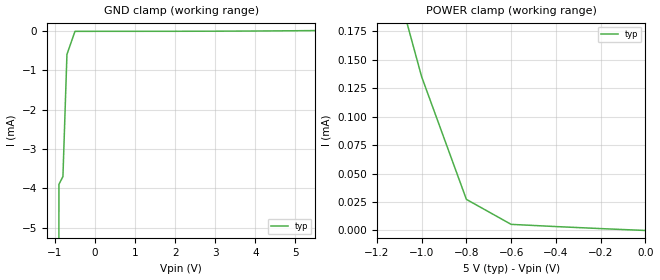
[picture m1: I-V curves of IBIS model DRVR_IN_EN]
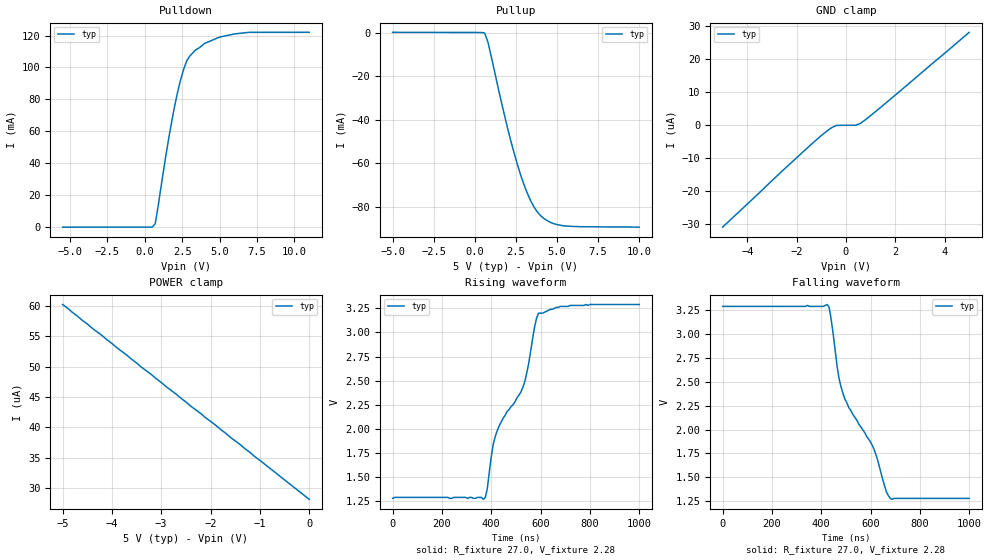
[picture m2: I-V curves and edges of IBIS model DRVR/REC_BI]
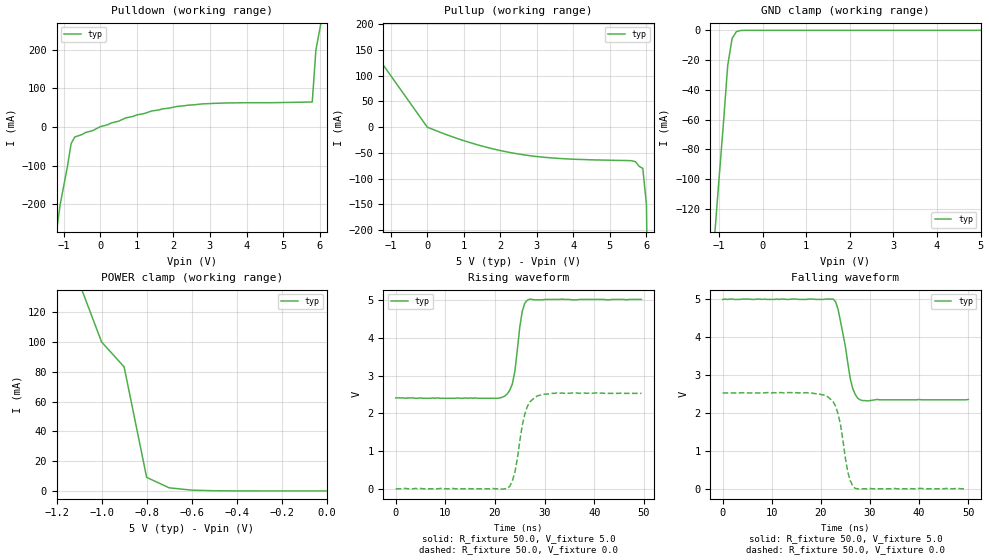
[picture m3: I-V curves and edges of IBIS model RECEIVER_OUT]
|   Texas Instruments Incorporated
|   Data Transmissions Products
|   IBIS Model for SN65HVD1786
|   SOIC 8-pin (D), PDIP 8-pin (P), VCC=5V
[IBIS Ver]   3.2
[Comment char]   |_char
[File name]   sllc356.ibs
[File Rev]   1.0
[Date]   6Aug08
[Source]   File originated at Texas Instruments Incorporated.
   Data Transmission Products Group.
[Notes]
[Disclaimer]
(C) Copyright Texas Instruments Incorporated 2002
   All rights reserved
  Texas Instruments Incorporated hereby grants the user of this IBIS
model a non-exclusive, nontransferable license to use this IBIS model
under the following terms.  Before using this IBIS model, the user
should read this license.  If the user does not accept these terms,
the IBIS model should be returned to Texas Instruments within 30 days.
  The user is granted this license only to use the IBIS model and
is not granted rights to sell, load, rent, lease or license the IBIS
model in whole or in part, or in modified form to anyone other than
user.  User may modify the IBIS model to suit its specific applications
but rights to derivative works and such modifications shall belong to
Texas Instruments.
  This IBIS model is provided on an "AS IS" basis and Texas Instruments
makes absolutely no warranty with respect to the information contained
herein.  TEXAS INSTRUMENTS DISCLAIMS AND CUSTOMER WAIVES ALL WARRANTIES,
EXPRESS OR IMPLIED, INCLUDING WARRANTIES OF MERCHANTABILITY OR FITNESS
FOR A PARTICULAR PURPOSE. The entire risk as to quality and performance
is with the Customer. ACCORDINGLY, IN NO EVENT SHALL THE COMPANY BE LIABLE
FOR ANY DAMAGES, WHETHER IN CONTRACT OR TORT,INCLUDING ANY LOST PROFITS
OR OTHER INCIDENTAL, CONSEQUENTIAL, EXEMPLARY, OR PUNITIVE DAMAGES ARISING
OUT OF THE USE OR APPLICATION OF THE IBIS model provided in this package.
Further, Texas Instruments reserves the right to discontinue or make changes
without notice to any product herein to improve reliability, function, or
design. Texas Instruments does not convey any license under patent rights
or any other intellectual property rights, including those of third parties.
Contact Texas Instruments at ATTN:DATA TRANSMISSIONS
[Copyright]   Copyright 2002, Texas Instruments, All Rights Reserved
[Component]   HVD1786_D
[Manufacturer]  Texas Instruments Incorporated
[Package]
|   typ   min   max
R_pkg   0.1017   0.0608   0.1359
L_pkg   1.9890nH   1.6927nH   2.3143nH
C_pkg   0.3794pF   0.3519pF   0.3977pF
[Pin]   signal_name   model_name   R_pin   L_pin   C_pin
1   R   RECEIVER_OUT   0.108   1.993n   0.363p
2   REB   DRVR_IN_EN   0.103   1.929n   0.373p
3   DE   DRVR_IN_EN   0.103   1.932n   0.373p
4   D   DRVR_IN_EN   0.107   2.016n   0.352p
5   GND   GND   0.064   1.778n   0.394p
6   A   DRVR/REC_BI   0.131   2.258n   0.391p
7   B   DRVR/REC_BI   0.136   2.314n   0.391p
8   VCC   POWER   0.061   1.693n   0.398p
[Diff_pin]   inv_pin   vdiff   tdelay_typ   tdelay_min   tdelay_max
| The 'A' pin is Diff_pin and the 'B' pin is the inv_pin
6   7   0.200   0   0   0
[Component]   HVD1786_P
[Manufacturer]  Texas Instruments Incorporated
[Package]
|   typ   min   max
R_pkg   0.0833   0.0374   0.1222
L_pkg   2.7019nH   1.3887nH   3.6744nH
C_pkg   0.6414pF   0.3892pF   0.8943pF
[Pin]   signal_name   model_name   R_pin   L_pin   C_pin
1   R   RECEIVER_OUT   0.078   3.269n   0.675p
2   REB   DRVR_IN_EN   0.100   2.510n   0.648p
3   DE   DRVR_IN_EN   0.111   2.858n   0.640p
4   D   DRVR_IN_EN   0.074   2.765n   0.640p
5   GND   GND   0.037   1.389n   0.389p
6   A   DRVR/REC_BI   0.105   3.674n   0.894p
7   B   DRVR/REC_BI   0.122   2.925n   0.663p
8   VCC   POWER   0.038   2.226n   0.583p
[Diff_pin]   inv_pin   vdiff   tdelay_typ   tdelay_min   tdelay_max
| The 'A' pin is Diff_pin and the 'B' pin is the inv_pin
6   7   0.200   0   0   0
| Models and submodels in the file (3): DRVR_IN_EN (Input), DRVR/REC_BI (I/O), RECEIVER_OUT (3-state)
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|   Driver Input / Receiver Enable Model
[Model]   DRVR_IN_EN
Model_type   Input
|Signals   D,DE,RE
Vinh = 2.0
Vinl = 0.8
|   typ   min   max
C_comp   1.0pF   NA   NA
|   typ   min   max
[Temperature Range]   25.0   -40   105
[Voltage range]   5.0V   4.5V   5.5V
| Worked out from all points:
|   GND clamp passes 1 mA (typ) near -0.71 V on its own axis
|   POWER clamp passes 1 mA (typ) near -2.08 V on its own axis
[GND_clamp]
|   Voltage   I(typ)   I(min)   I(max)
-5.5V     -8.7A      NA         NA
-2V       -1.9A      NA         NA
-900mV    -3.9mA     NA         NA
-800mV    -3.7mA     NA         NA
-700mV    -600uA     NA         NA
-500mV    -16uA      NA         NA
5.5V      4.37uA     NA         NA
[Power_clamp]
| Note that the[POWER_clamp]voltage table is referenced to Vcc
| and is calculated using Vtable=Vcc - Vmeasured.
|   Voltage   I(typ)   I(min)   I(max)
-5.5V     4.1mA      NA         NA
-1.2V     279uA      NA         NA
-1V       135uA      NA         NA
-800mV    27.3uA     NA         NA
-600mV    5.38uA     NA         NA
0V        8.71nA     NA         NA
|   Driver Output / Receiver Input Model
[Model]   DRVR/REC_BI
Model_type   I/O
| Signals   A,B
Vinl = 0.9V
Vinh = 2.8V
Vmeas = 1.7V   |Reference voltage for timing measurements
Cref = 50pF   |Timing specification test load capacitance value
Rref = 54   |Note: 54 Ohm load; single-ended configuration
|   Timing specification test load voltage
| variable   typ   min   max
C_comp   1.0pF   NA   NA
|   typ   min   max
[Temperature Range]   25.0   -40   105
[Voltage range]   5.0V   4.5V   5.5V
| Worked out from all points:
|   slope of the pulldown table from 0 to 0.75 V, typ, clamps not added: 149 ohm
|   slope of the pullup table from 0 to 0.75 V, typ, clamps not added: 222 ohm
|   rising waveform, R_fixture 27.0, V_fixture 2.28: 20-80 % time 166ns typ, NA min, NA max; typ from 1.28 V to 3.29 V
|   falling waveform, R_fixture 27.0, V_fixture 2.28: 20-80 % time 175ns typ, NA min, NA max; typ from 3.29 V to 1.28 V
[Pulldown]
|   Voltage   I(typ)   I(min)   I(max)
-5.5V     -52uA      NA         NA
500mV     -6.84uA    NA         NA
700mV     2.18mA     NA         NA
1.6V      55.5mA     NA         NA
2.2V      84.7mA     NA         NA
2.4V      92.4mA     NA         NA
2.8V      104mA      NA         NA
3.4V      111mA      NA         NA
4V        115mA      NA         NA
5V        119mA      NA         NA
6V        121mA      NA         NA
11V       122mA      NA         NA
[Pullup]
|   Voltage   I(typ)   I(min)   I(max)
| Note that the[Pullup]voltage table is referenced to Vcc
| and is calculated using Vtable=Vcc - Vmeasured.
-5V       147uA      NA         NA
600mV     -176uA     NA         NA
800mV     -4.36mA    NA         NA
2V        -44mA      NA         NA
2.6V      -60.7mA    NA         NA
3V        -69.9mA    NA         NA
3.2V      -73.7mA    NA         NA
3.4V      -77.1mA    NA         NA
3.8V      -82.2mA    NA         NA
4.4V      -86.2mA    NA         NA
5.4V      -88.6mA    NA         NA
10V       -89.2mA    NA         NA
[GND_clamp]
|   Voltage   I(typ)   I(min)   I(max)
| Outputs in High Impedance (off)
-5V       -30.9uA    NA         NA
-2.5V     -13.3uA    NA         NA
-800mV    -1.92uA    NA         NA
-400mV    -75.6nA    NA         NA
400mV     10.5nA     NA         NA
600mV     616nA      NA         NA
1.6V      6.63uA     NA         NA
5V        28.2uA     NA         NA
[POWER_clamp]
|   Voltage   I(typ)   I(min)   I(max)
| Note that the [POWER_clamp] voltage table is referenced to Vcc
| and is calculated using Vtable = Vcc - Vmeasured.
| Outputs in Tri-state.
-5V       60.2uA     NA         NA
-4.4V     56.3uA     NA         NA
-4.2V     55.1uA     NA         NA
0V        28.2uA     NA         NA
[Ramp]
|   typ   min   max
dV/dt_r   1.50V/177.7ns   NA   NA
dV/dt_f   1.50V/199.9ns   NA   NA
R_load = 27ohm | Note: The measurement is on a single-ended configuration
|   with 54ohm line-to-line.
[Rising Waveform]
R_fixture = 27.0
V_fixture = 2.28
C_fixture = 0p
L_fixture = 0n
|   V(typ)   V(min)   V(max)
0s        1.28V      NA         NA
368ns     1.27V      NA         NA
384ns     1.38V      NA         NA
400ns     1.71V      NA         NA
416ns     1.92V      NA         NA
528ns     2.43V      NA         NA
552ns     2.68V      NA         NA
576ns     3.06V      NA         NA
592ns     3.2V       NA         NA
1us       3.29V      NA         NA
[Falling Waveform]
R_fixture = 27.0
V_fixture = 2.28
C_fixture = 0p
L_fixture = 0n
|   V(typ)   V(min)  V(max)
0s        3.29V      NA         NA
424ns     3.31V      NA         NA
432ns     3.28V      NA         NA
472ns     2.54V      NA         NA
488ns     2.38V      NA         NA
512ns     2.23V      NA         NA
608ns     1.83V      NA         NA
664ns     1.35V      NA         NA
680ns     1.28V      NA         NA
1us       1.28V      NA         NA
|   Receiver Output Model
[Model]   RECEIVER_OUT
Model_type   3-state
| Signals   R
Vmeas = 2.2V   |Reference voltage for timing measurements
Cref = 15pF   |Timing specification test load capacitance value
Vref = 0   |Timing specification test load voltage; GND
| variable   typ   min   max
C_comp   1.0pF   NA   NA
|   typ   min   max
[Temperature Range]   25.0   -40   105
[Voltage range]   5.0V   4.5V   5.5V
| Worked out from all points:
|   slope of the pulldown table from 0 to 0.75 V, typ, clamps not added: 31.8 ohm
|   slope of the pullup table from 0 to 0.75 V, typ, clamps not added: 36.9 ohm
|   GND clamp passes 1 mA (typ) near -0.60 V on its own axis
|   POWER clamp passes 1 mA (typ) near -0.63 V on its own axis
|   rising waveform, R_fixture 50.0, V_fixture 5.0: 20-80 % time 1.52ns typ, NA min, NA max; typ from 2.41 V to 5.01 V
|   falling waveform, R_fixture 50.0, V_fixture 5.0: 20-80 % time 2.09ns typ, NA min, NA max; typ from 4.99 V to 2.36 V
|   rising waveform, R_fixture 50.0, V_fixture 0.0: 20-80 % time 2.01ns typ, NA min, NA max; typ from 0.01 V to 2.53 V
|   falling waveform, R_fixture 50.0, V_fixture 0.0: 20-80 % time 2.01ns typ, NA min, NA max; typ from 2.53 V to 0.01 V
[Pulldown]
|   Voltage   I(typ)   I(min)  I(max)
-5V       -2.8A      NA         NA
-2.1V     -900mA     NA         NA
-1.1V     -200mA     NA         NA
-900mV    -101mA     NA         NA
-800mV    -42.3mA    NA         NA
-700mV    -25.5mA    NA         NA
700mV     24mA       NA         NA
2.8V      60.2mA     NA         NA
5.8V      65mA       NA         NA
5.9V      200mA      NA         NA
6.1V      300mA      NA         NA
10V       12A        NA         NA
[Pullup]
|   Voltage   I(typ)   I(min)  I(max)
| Note that the[Pullup]voltage table is referenced to Vcc
| and is calculated using Vtable=Vcc - Vmeasured.
-5V       500mA      NA         NA
-2V       200mA      NA         NA
-1V       100mA      NA         NA
0V        57uA       NA         NA
1.4V      -34.8mA    NA         NA
2.6V      -53.3mA    NA         NA
3.6V      -60.7mA    NA         NA
5.7V      -67.1mA    NA         NA
5.9V      -80mA      NA         NA
6V        -150mA     NA         NA
7V        -5.5A      NA         NA
10V       -22.5A     NA         NA
[GND_clamp]
|   Voltage   I(typ)   I(min)   I(max)
| Outputs in High Impedance (off)
-5V       -1.7A      NA         NA
-2V       -480mA     NA         NA
-1V       -100mA     NA         NA
-900mV    -63.1mA    NA         NA
-800mV    -23.5mA    NA         NA
-700mV    -5.53mA    NA         NA
-600mV    -837uA     NA         NA
-400mV    -4.64uA    NA         NA
5V        91.2pA     NA         NA
[POWER_clamp]
|   Voltage   I(typ)   I(min)   I(max)
| Note that the [POWER_clamp] voltage table is referenced to Vcc
| and is calculated using Vtable = Vcc - Vmeasured.
| Outputs in Tri-state.
-5V       1.7A       NA         NA
-2V       500mA      NA         NA
-1V       100mA      NA         NA
-900mV    83.3mA     NA         NA
-800mV    9.11mA     NA         NA
-700mV    2.08mA     NA         NA
-600mV    537uA      NA         NA
-500mV    126uA      NA         NA
0V        91.2pA     NA         NA
[Ramp]
|   typ   min   max
dV/dt_r   1.70V/1477ps   NA   NA
dV/dt_f   1.50V/1948ps   NA   NA
R_load = 50
[Rising Waveform]
R_fixture = 50.0
V_fixture = 5.0
V_fixture_min = 4.5
V_fixture_max = 5.5
C_fixture = 0p
L_fixture = 0n
|   V(typ)   V(min)  V(max)
0s        2.41V      NA         NA
20.5ns    2.4V       NA         NA
22ns      2.46V      NA         NA
23.5ns    2.78V      NA         NA
24ns      3.11V      NA         NA
25ns      4.29V      NA         NA
25.5ns    4.7V       NA         NA
26ns      4.91V      NA         NA
27ns      5.02V      NA         NA
49.5ns    5.01V      NA         NA
[Falling Waveform]
R_fixture = 50.0
V_fixture = 5.0
V_fixture_min = 4.5
V_fixture_max = 5.5
C_fixture = 0p
L_fixture = 0n
|   V(typ)   V(min)  V(max)
0s        4.99V      NA         NA
22.5ns    5V         NA         NA
23ns      4.93V      NA         NA
23.5ns    4.73V      NA         NA
25ns      3.74V      NA         NA
26ns      2.89V      NA         NA
26.5ns    2.64V      NA         NA
27.5ns    2.39V      NA         NA
29.5ns    2.32V      NA         NA
50ns      2.36V      NA         NA
[Rising Waveform]
R_fixture = 50.0
V_fixture = 0.0
C_fixture = 0p
L_fixture = 0n
|   V(typ)   V(min)  V(max)
0s        10mV       NA         NA
22.5ns    20mV       NA         NA
23ns      80mV       NA         NA
24ns      440mV      NA         NA
25.5ns    1.69V      NA         NA
26ns      1.98V      NA         NA
27ns      2.3V       NA         NA
28ns      2.42V      NA         NA
32.5ns    2.54V      NA         NA
49.5ns    2.53V      NA         NA
[Falling Waveform]
R_fixture = 50.0
V_fixture = 0.0
C_fixture = 0p
L_fixture = 0n
|   V(typ)   V(min)  V(max)
0s        2.53V      NA         NA
17ns      2.54V      NA         NA
21.5ns    2.42V      NA         NA
22.5ns    2.3V       NA         NA
23.5ns    1.98V      NA         NA
24ns      1.69V      NA         NA
25.5ns    440mV      NA         NA
26.5ns    80mV       NA         NA
27ns      20mV       NA         NA
49.5ns    10mV       NA         NA
